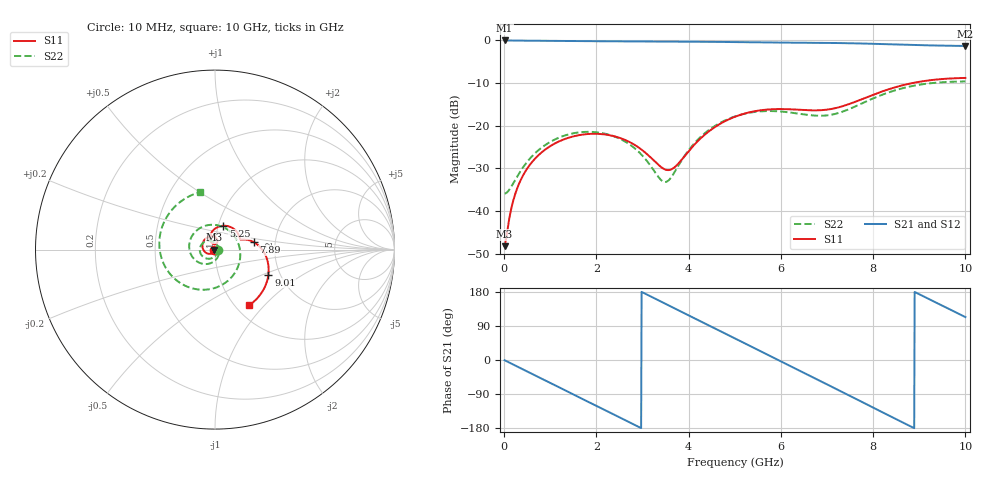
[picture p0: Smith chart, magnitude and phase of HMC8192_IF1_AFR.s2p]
! Analog Devices, Inc.
! 1 Analog Way
! Wilmington, MA 01887
! http://www.analog.com
! Date:  2021-09-17 NN
! Board Name:  EVALHMC8192LG Revision A with HMC8192LG installed
! File Description:  Automatic Fixture Removal S-Parameters for IF1 Port connector and board loss de-embedding
! File Generation:  Calibrated Network Analyzer
! Chip Part Number:  HMC8192
! Chip Description:  Wideband IQ Mixer
! Chip Frequency:  20 to 42 GHz
! Chip Package:  LGA_CAV, 4 x 4 x 1.55 mm
! IF1 Port:  HMC8192LG removed and end of trace left open
! Note:
!  Analog Devices supplies this data as a sample of measured data at the evaluation board
!  ports for this product.  Your particular data for this product may vary.
!  Analog Devices reserves the right to change this data at anytime.
!  All lines below in this file are as is from the Network Analyzer.
!Agilent Technologies,N5245A,MY52451809,A.10.47.06
!Automatic Fixture Removal (AFR)
!Date: Friday, September 17, 2021 2:57:08 AM
!S2P File: Measurements: S11,S21,S12,S22:
# MHz S  RI  R 50
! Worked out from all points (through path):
!   1000 points, 10 MHz to 10 GHz, reference 50 ohm
!   highest |S21| = 0.01 dB at 10 MHz (marker M1); lowest = -1.3 dB at 10 GHz (marker M2)
!   group delay of S21, straight-line fit = 169 ps
!   lowest |S11| = -48.3 dB at 10 MHz (marker M3), VSWR 1.01, Z = 49.6 - j0.059 ohm
!   |S11| at or under -10 dB: start of sweep to 8.846 GHz
!   |S22| runs from -35.9 to -9.6 dB; largest |S21 - S12| = 1.4e-15
!   S11 on the Smith chart (normalised r, x): 10 MHz: 0.99, -0.00; 5.25 GHz: 1.06, +0.29; 7.89 GHz: 1.54, +0.14; 9.01 GHz: 1.74, -0.54; 10 GHz: 1.16, -0.83
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10  -0.00382 -0.000595  1.001 -0.0106  1.001 -0.0106  0.016 -0.000848
240  -0.00847 -0.0134  0.9659 -0.2511  0.9659 -0.2511  0.012 -0.0198
530  -0.024 -0.0231  0.842 -0.5296  0.842 -0.5296  -0.00255 -0.0394
1130  -0.063 -0.00436  0.3619 -0.9193  0.3619 -0.9193  -0.0509 -0.0485
1680  -0.0656 0.0431  -0.1998 -0.9622  -0.1998 -0.9622  -0.0828 -0.0156
2100  -0.0393 0.0696  -0.5908 -0.7818  -0.5908 -0.7818  -0.0799 0.0203
2570  -0.00249 0.0699  -0.8897 -0.4061  -0.8897 -0.4061  -0.0487 0.0469
2960  0.0135 0.0517  -0.9767 -0.0158  -0.9767 -0.0158  -0.0128 0.0451
3340  0.00854 0.0339  -0.9036 0.3675  -0.9036 0.3675  0.0152 0.0202
3570  -0.00205 0.0301  -0.787 0.5741  -0.787 0.5741  0.0228 -0.00323
4210  -0.028 0.0608  -0.2503 0.9353  -0.2503 0.9353  -0.0105 -0.0689
4600  -0.0183 0.0972  0.1454 0.952  0.1454 0.952  -0.0633 -0.0799
5010  0.0179 0.1266  0.528 0.7981  0.528 0.7981  -0.119 -0.0496
5250  0.0463 0.1329  0.7084 0.6383  0.7084 0.6383  -0.1391 -0.0136
5960  0.1181 0.1034  0.945 -0.014  0.945 -0.014  -0.0979 0.1102
6670  0.1386 0.0613  0.676 -0.6534  0.676 -0.6534  0.0588 0.1187
7290  0.1567 0.0563  0.1281 -0.9238  0.1281 -0.9238  0.141 -0.026
7890  0.2149 0.042  -0.4459 -0.8027  -0.4459 -0.8027  0.0479 -0.1912
8340  0.2681 -0.00767  -0.7541 -0.4975  -0.7541 -0.4975  -0.1129 -0.2191
9010  0.2976 -0.1389  -0.875 0.1093  -0.875 0.1093  -0.3008 -0.0376
9460  0.2659 -0.2306  -0.7207 0.4893  -0.7207 0.4893  -0.2814 0.1584
10000  0.1912 -0.3097  -0.3403 0.7927  -0.3403 0.7927  -0.0853 0.3197
